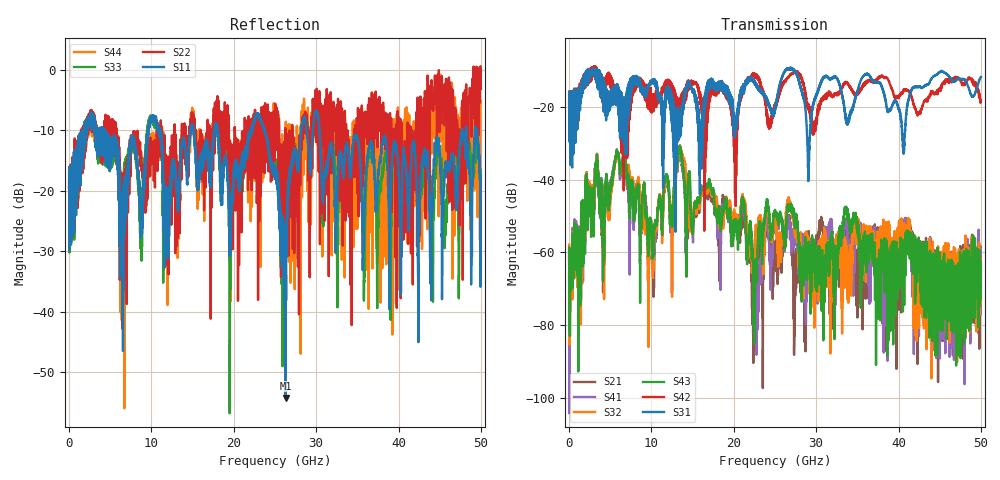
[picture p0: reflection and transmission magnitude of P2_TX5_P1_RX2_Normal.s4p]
!Keysight Technologies,N5225B,MY57041031,A.13.20.10
!Date: Friday, May 31, 2019 11:16:37
!Correction: S11(Full 4 Port(1,2,3,4))
!S12(Full 4 Port(1,2,3,4))
!S13(Full 4 Port(1,2,3,4))
!S14(Full 4 Port(1,2,3,4))
!S21(Full 4 Port(1,2,3,4))
!S22(Full 4 Port(1,2,3,4))
!S23(Full 4 Port(1,2,3,4))
!S24(Full 4 Port(1,2,3,4))
!S31(Full 4 Port(1,2,3,4))
!S32(Full 4 Port(1,2,3,4))
!S33(Full 4 Port(1,2,3,4))
!S34(Full 4 Port(1,2,3,4))
!S41(Full 4 Port(1,2,3,4))
!S42(Full 4 Port(1,2,3,4))
!S43(Full 4 Port(1,2,3,4))
!S44(Full 4 Port(1,2,3,4))
!S4P File: Measurements: <S11,S12,S13,S14>,
!<S21,S22,S23,S24>,
!<S31,S32,S33,S34>,
!<S41,S42,S43,S44>:
# Hz S  dB  R 50.0
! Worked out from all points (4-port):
!   5000 points, 10 MHz to 50 GHz, reference 50 ohm
!   strongest paths, dB at 10 MHz, 12.51 GHz, 25.01 GHz, 37.51 GHz, 50 GHz:
!     S31: -19.5, -17.8, -20.9, -13.2, -11.7
!     S42: -19.3, -16.2, -19.3, -12.1, -18.0
!     S43: -58.7, -51.3, -49.2, -65.0, -63.2
!     S32: -57.9, -72.2, -50.3, -57.9, -69.6
!     S41: -60.7, -50.6, -52.8, -65.0, -64.8
!     S21: -65.8, -65.7, -58.2, -56.7, -69.6
!   lowest |S11| = -54.2 dB at 26.29 GHz (marker M1), VSWR 1.00, Z = 50.1 - j0.188 ohm
!   |S11| at or under -10 dB: 4.282 GHz to 9.568 GHz (5.286 GHz wide, 76.3 % of centre); 23.74 GHz to 28.18 GHz (4.441 GHz wide, 17.1 % of centre); 30.39 GHz to 47.7 GHz (17.32 GHz wide, 44.3 % of centre)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
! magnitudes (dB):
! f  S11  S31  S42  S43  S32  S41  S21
! 10 MHz  -19.8  -19.5  -19.3  -58.7  -57.9  -60.7  -65.8
! 5.81 GHz  -15.7  -14.8  -17.6  -31.9  -32.4  -32.2  -32.6
! 9.67 GHz  -9.2  -14.0  -16.2  -60.1  -66.9  -56.9  -70.4
! 13.51 GHz  -15.1  -22.1  -21.9  -31.2  -30.9  -32.6  -32.3
! 26.29 GHz  -54.2  -9.7  -12.8  -55.0  -50.9  -55.6  -55.4
! 30.01 GHz  -6.8  -16.7  -23.8  -61.2  -68.5  -59.4  -57.9
! 50 GHz  -19.2  -11.7  -18.0  -63.2  -69.6  -64.8  -69.6
